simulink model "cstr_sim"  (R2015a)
settings: Solver=ode45  StartTime=0.0  StopTime=10  RelTol=1e-3
StopFcn:
  | plot_reactor
libraries: simulink x5, realtime_pacer_lib x1

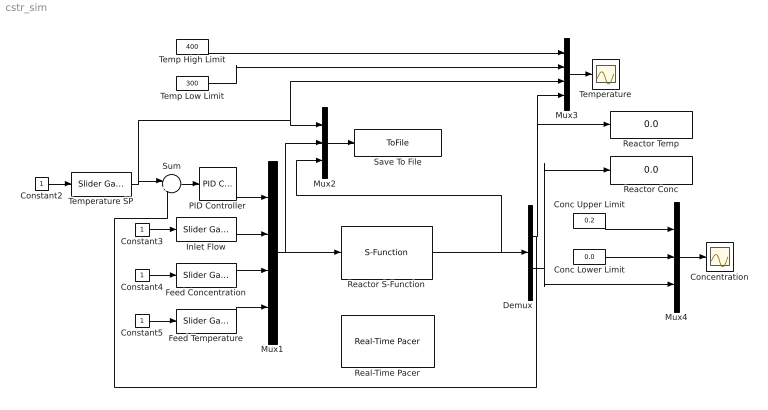
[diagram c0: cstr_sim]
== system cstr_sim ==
  Conc Lower Limit : Constant  Value=0.0
  Conc Upper Limit : Constant  Value=0.2
  Concentration : Scope
  Constant{2..5} (4 alike) : Constant
  Demux : Demux  Outputs=2
  Feed Concentration : simulink/Math Operations/Slider Gain  low=0  gain=1  high=1
  Feed Temperature : simulink/Math Operations/Slider Gain  low=300  gain=350  high=400
  Inlet Flow : simulink/Math Operations/Slider Gain  low=0  gain=100  high=200
  Mux1 : Mux
  Mux2 : Mux  Inputs=3
  Mux3 : Mux
  Mux4 : Mux  Inputs=3
  PID Controller : simulink/Continuous/PID Controller  Controller=PID  TimeDomain=Continuous-time  SampleTime=-1  IntegratorMethod=Forward Euler  FilterMethod=Forward Euler  Form=Parallel  UseFilter=on  ControllerParametersSource=internal  P=1  I=1  D=0  N=100  InitialConditionSource=internal  InitialConditionForIntegrator=280  InitialConditionForFilter=0  ExternalReset=none  LimitOutput=on  UpperSaturationLimit=350  LowerSaturationLimit=250  LinearizeAsGain=on  AntiWindupMode=clamping  Kb=1  TrackingMode=off  Kt=1  PParamMin=[]  PParamMax=[]  IParamMin=[]  IParamMax=[]  DParamMin=[]  DParamMax=[]  NParamMin=[]  NParamMax=[]  KbParamMin=[]  KbParamMax=[]  KtParamMin=[]  KtParamMax=[]  POutMin=[]  POutMax=[]  IOutMin=[]  IOutMax=[]  DOutMin=[]  DOutMax=[]  NOutMin=[]  NOutMax=[]  KbOutMin=[]  KbOutMax=[]  KtOutMin=[]  KtOutMax=[]  IntegratorOutMin=[]  IntegratorOutMax=[]  FilterOutMin=[]  FilterOutMax=[]  SumOutMin=[]  SumOutMax=[]  SumI1OutMin=[]  SumI1OutMax=[]  SumI2OutMin=[]  SumI2OutMax=[]  SumI3OutMin=[]  SumI3OutMax=[]  SumDOutMin=[]  SumDOutMax=[]  SaturationOutMin=[]  SaturationOutMax=[]  IntegratorContinuousStateAttributes=''  IntegratorStateMustResolveToSignalObject=off  IntegratorRTWStateStorageClass=Auto  FilterContinuousStateAttributes=''  FilterStateMustResolveToSignalObject=off  FilterRTWStateStorageClass=Auto  DifferentiatorICPrevScaledInput=0  DifferentiatorOutMin=[]  DifferentiatorOutMax=[]
  Reactor Conc : Display
  Reactor S-Function : S-Function  FunctionName=reactor
  Reactor Temp : Display
  Real-Time Pacer : realtime_pacer_lib/Real-Time Pacer  simTimePerRealTime=1/5
  Save To File : ToFile  Filename=data.mat  MatrixName=cstr  SampleTime=0.05
  Sum : Sum  Inputs=|+-
  Temp High Limit : Constant  Value=400
  Temp Low Limit : Constant  Value=300
  Temperature : Scope
  Temperature SP : simulink/Math Operations/Slider Gain  low=300  gain=320  high=400
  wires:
  Reactor S-Function/1 -> Mux2/3, Demux/1
  Constant3/1 -> Inlet Flow/1
  Mux2/1 -> Save To File/1
  Mux1/1 -> Mux2/2, Reactor S-Function/1
  Inlet Flow/1 -> Mux1/2
  PID Controller/1 -> Mux1/1
  Constant2/1 -> Temperature SP/1
  Demux/2 -> Mux4/3, Reactor Conc/1
  Constant4/1 -> Feed Concentration/1
  Feed Concentration/1 -> Mux1/3
  Constant5/1 -> Feed Temperature/1
  Feed Temperature/1 -> Mux1/4
  Demux/1 -> Sum/2, Mux3/4, Reactor Temp/1
  Temp High Limit/1 -> Mux3/1
  Temp Low Limit/1 -> Mux3/2
  Mux3/1 -> Temperature/1
  Conc Upper Limit/1 -> Mux4/1
  Conc Lower Limit/1 -> Mux4/2
  Mux4/1 -> Concentration/1
  Sum/1 -> PID Controller/1
  Temperature SP/1 -> Mux3/3, Mux2/1, Sum/1
